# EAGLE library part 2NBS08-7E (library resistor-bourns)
BOURNS RESISTOR NETWORK
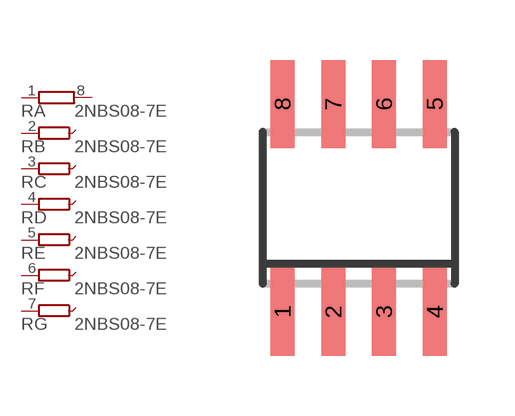
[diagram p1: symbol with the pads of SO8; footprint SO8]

Designator prefix R; gates A=R1NV0 B=R1NVXX C=R1NVXX D=R1NVXX E=R1NVXX F=R1NVXX G=R1NVXX

## 2NBS08-7E (OC_FARNELL: unknown; OC_NEWARK: unknown)  [SO8]
1  A:1  pas
2  B:1  pas
3  C:1  pas
4  D:1  pas
5  E:1  pas
6  F:1  pas
7  G:1  pas
8  A:2  pas

## Footprint SO8 (pad centres in mm)
BOURNS RESISTOR NETWORK
smd 0.6 x 2.2: 1 -1.905,-2.6; 2 -0.635,-2.6; 3 0.635,-2.6; 4 1.905,-2.6; 5 1.905,2.6; 6 0.635,2.6; 7 -0.635,2.6; 8 -1.905,2.6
